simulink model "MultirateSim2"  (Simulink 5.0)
settings: Solver=ode45  StartTime=0.0  StopTime=20  RelTol=1e-3
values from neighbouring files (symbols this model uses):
  AL = A^L    [Multirate.m]
  BL = [A^i*B,BL]    [Multirate.m]
  CL = [CL;C*A^i]    [Multirate.m]
  DL = zeros(L,L)    [Multirate.m]
undefined symbols (not defined in the file or in its folder): denDc, numDc

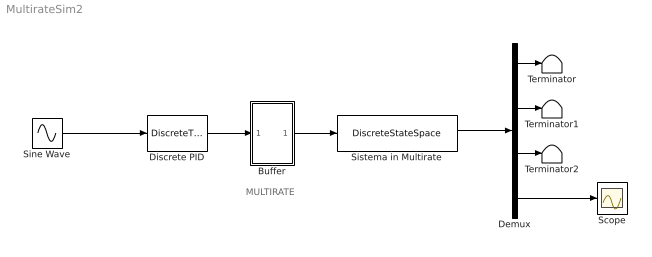
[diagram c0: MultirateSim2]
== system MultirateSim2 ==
  note: MULTIRATE
  Buffer : Subsystem
  Demux : Demux
  Discrete PID : DiscreteTransferFcn  Numerator=numDc  Denominator=denDc  SampleTime=0.004
  Scope : Scope
  Sine Wave : Sin  Frequency=10  SampleTime=0.016
  Sistema in Multirate : DiscreteStateSpace  A=AL  B=BL  C=CL  D=DL  SampleTime=0.016
  Terminator : Terminator
  Terminator1 : Terminator
  Terminator2 : Terminator
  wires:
  Sine Wave/1 -> Discrete PID/1
  Discrete PID/1 -> Buffer/1(In1)
  Buffer/1(Out1) -> Sistema in Multirate/1
  Sistema in Multirate/1 -> Demux/1
  Demux/4 -> Scope/1
  Demux/1 -> Terminator/1
  Demux/2 -> Terminator1/1
  Demux/3 -> Terminator2/1

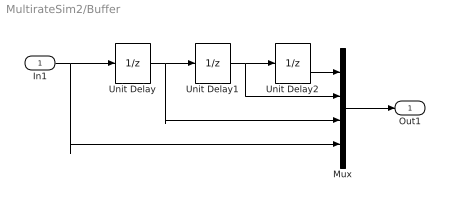
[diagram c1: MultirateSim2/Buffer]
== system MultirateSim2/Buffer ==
  In1 : Inport
  Mux : Mux
  Unit Delay : UnitDelay  SampleTime=-1
  Unit Delay1 : UnitDelay  SampleTime=-1
  Unit Delay2 : UnitDelay  SampleTime=-1
  Out1 : Outport
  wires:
  Unit Delay/1 -> Unit Delay1/1, Mux/3
  Unit Delay1/1 -> Unit Delay2/1, Mux/2
  In1/1 -> Mux/4, Unit Delay/1
  Unit Delay2/1 -> Mux/1
  Mux/1 -> Out1/1
